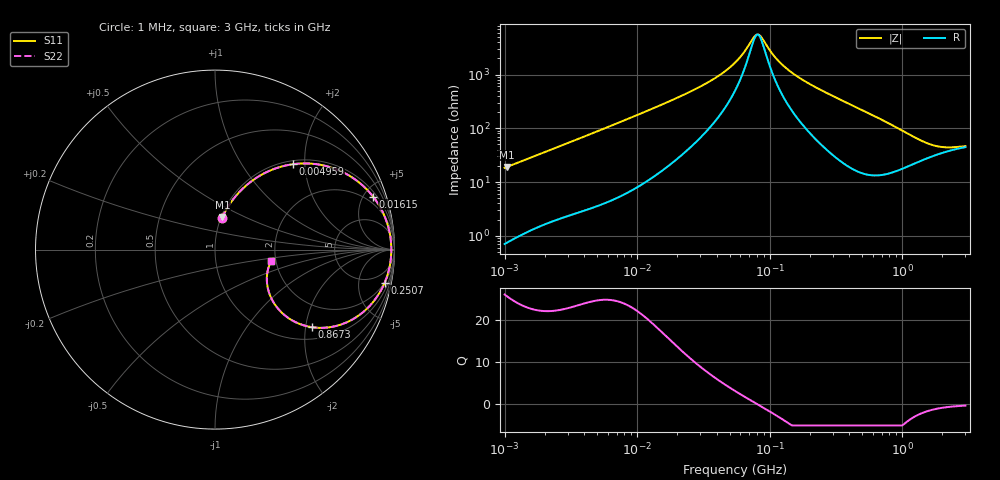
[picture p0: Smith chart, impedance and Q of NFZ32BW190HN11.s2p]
! NFZ32BW190HN11
# Hz S RI R 50
!Freq.(Hz) S11(Real) S11(Imag) S21(Real) S21(Imag) S12(Real) S12(Imag) S22(Real) S22(Imag)
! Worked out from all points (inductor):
!   401 points, 1 MHz to 3 GHz, reference 50 ohm
!   read as one part in series: L = 2.9 uH near 1.041 MHz
!   highest Q = 25.6 at 1.041 MHz (marker M1), where L = 2.91 uH
!   self-resonance near 81.14 MHz
!   S11 on the Smith chart (normalised r, x): 1 MHz: 1.01, +0.37; 4.959 MHz: 1.07, +1.74; 16.15 MHz: 1.35, +5.82; 250.7 MHz: 2, -10; 867.3 MHz: 1.31, -2.17; 3 GHz: 1.89, -0.26
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1000000  0.0388 0.175  0.9612 -0.175  0.9612 -0.175  0.0388 0.175
1040844  0.0417 0.1813  0.9583 -0.1813  0.9583 -0.1813  0.0417 0.1813
2097170  0.1345 0.3193  0.8655 -0.3193  0.8655 -0.3193  0.1345 0.3193
3823119  0.319 0.4455  0.681 -0.4455  0.681 -0.4455  0.319 0.4455
4959344  0.4336 0.4757  0.5664 -0.4757  0.5664 -0.4757  0.4336 0.4757
7858845  0.6496 0.4567  0.3504 -0.4567  0.3504 -0.4567  0.6496 0.4567
1.461624e7  0.8592 0.3208  0.1408 -0.3208  0.1408 -0.3208  0.8592 0.3208
1.615473e7  0.8804 0.2955  0.1196 -0.2955  0.1196 -0.2955  0.8804 0.2955
3.456417e7  0.9646 0.1294  0.0354 -0.1294  0.0354 -0.1294  0.9646 0.1294
5.477226e7  0.9792 0.0552  0.0208 -0.0552  0.0208 -0.0552  0.9792 0.0552
7.544761e7  0.9823 0.01  0.0177 -0.01  0.0177 -0.01  0.9823 0.01
8.173662e7  0.9824 -0.00101  0.0176 0.00101  0.0176 0.00101  0.9824 -0.00101
8.679508e7  0.9823 -0.00928  0.0177 0.00928  0.0177 0.00928  0.9823 -0.00928
1.244416e8  0.9786 -0.0605  0.0214 0.0605  0.0214 0.0605  0.9786 -0.0605
2.094008e8  0.9588 -0.1487  0.0412 0.1487  0.0412 0.1487  0.9588 -0.1487
2.507343e8  0.9449 -0.1858  0.0551 0.1858  0.0551 0.1858  0.9449 -0.1858
4.66327e8  0.8331 -0.3416  0.1669 0.3416  0.1669 0.3416  0.8331 -0.3416
8.005644e8  0.5876 -0.4361  0.4124 0.4361  0.4124 0.4361  0.5876 -0.4361
8.672962e8  0.5408 -0.4325  0.4592 0.4325  0.4592 0.4325  0.5408 -0.4325
1.488926e9  0.3089 -0.2608  0.6911 0.2608  0.6911 0.2608  0.3089 -0.2608
2.050964e9  0.2898 -0.1418  0.7102 0.1418  0.7102 0.1418  0.2898 -0.1418
3e9  0.3141 -0.0622  0.6859 0.0622  0.6859 0.0622  0.3141 -0.0622
